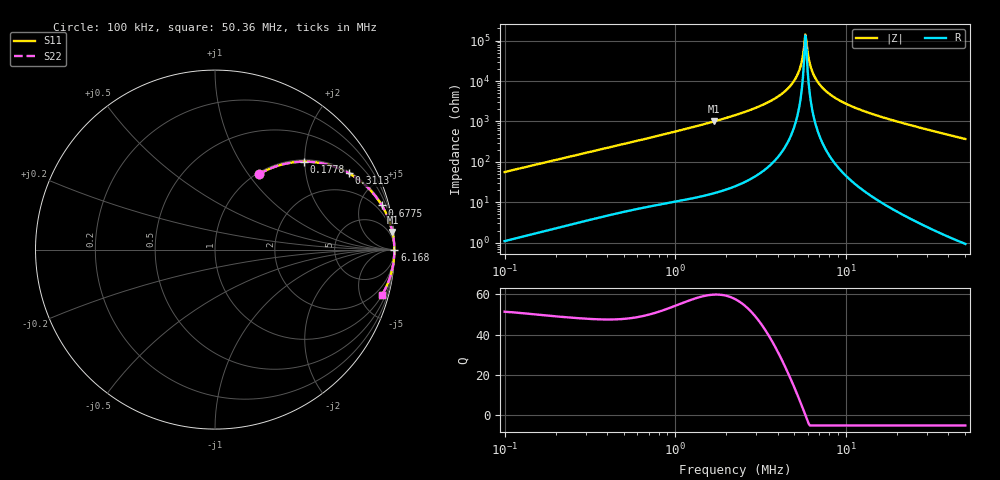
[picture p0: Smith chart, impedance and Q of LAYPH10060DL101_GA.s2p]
! LAYPH10060DL101_GA  S-PARAMETER MODEL  ( General Type )
! Model Generated by TAIYO YUDEN Corporation (http://www.ty-top.com)
! Version 3.0
! TAIYO YUDEN Control No. 180828NI43SB-FBB
! Copyright(c) 2017 TAIYO YUDEN CO.,LTD. All Rights Reserved.
! Product Description (link to TY-COMPAS)
! https://ds.yuden.co.jp/TYCOMPAS/or/detail?pn=LAYPH10060DL101MGA&u=M
! Products Name : Inductors
! Characteristics :
!  Inductance : 100 uH , SRF(min) : -Hz , DC Resistance(max) : 0.203 Ohm
!  Rated Current : Saturation :1.4 A , Temp Rise : 0.93 A (25 degC)
!  Case Size : 10.1 x 10.0 / 0.398 x 0.394 [mm/inch] , Thickness : 6 / 0.236 [mm/inch]
!  (Conditions: Temperature = 25 degC , DC Bias Current/Voltage = 0A / 0V)
! External Node Assignments :
!  1  o---GGG---o  2
! GND o---------o GND
! Frequency Range : 0.1MHz  -  50.361429MHz  [ 402 STEP ]
# MHz S RI R 50
! Freq[MHz].  S11 Real  S11 Imag  S21 Real  S21 Imag  S12 Real  S12 Imag  S22 Real  S22 Imag
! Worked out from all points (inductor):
!   401 points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, 100 kHz to 50.36 MHz, reference 50 ohm
!   read as one part in series: L = 89.2 uH near 103.2 kHz
!   highest Q = 59.7 at 1.696 MHz (marker M1), where L = 94.4 uH
!   self-resonance near 5.796 MHz
!   S11 on the Smith chart (normalised r, x): 100 kHz: 1.02, +1.12; 177.8 kHz: 1.04, +1.99; 311.3 kHz: 1.07, +3.46; 677.5 kHz: 1.15, +7.52; 6.168 MHz: open; 50.36 MHz: 1.02, -7.37
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0.1  0.2445 0.4202  0.7555 -0.4202  0.7555 -0.4202  0.2445 0.4202
0.177805  0.497 0.49  0.503 -0.49  0.503 -0.49  0.497 0.49
0.283532  0.7094 0.4437  0.2906 -0.4437  0.2906 -0.4437  0.7094 0.4437
0.311267  0.7452 0.4254  0.2548 -0.4254  0.2548 -0.4254  0.7452 0.4254
0.677478  0.9297 0.2457  0.0703 -0.2457  0.0703 -0.2457  0.9297 0.2457
0.803902  0.9488 0.2109  0.0512 -0.2109  0.0512 -0.2109  0.9488 0.2109
1.696112  0.9886 0.0981  0.0114 -0.0981  0.0114 -0.0981  0.9886 0.0981
2.279315  0.9942 0.068  0.00585 -0.068  0.00585 -0.068  0.9942 0.068
3.523312  0.9981 0.0331  0.00193 -0.0331  0.00193 -0.0331  0.9981 0.0331
4.589763  0.999 0.0152  0.000953 -0.0152  0.000953 -0.0152  0.999 0.0152
5.279436  0.9993 0.00616  0.000722 -0.00616  0.000722 -0.00616  0.9993 0.00616
5.446255  0.9993 0.00418  0.000694 -0.00418  0.000694 -0.00418  0.9993 0.00418
5.70642  0.9993 0.00122  0.000668 -0.00122  0.000668 -0.00122  0.9993 0.00122
5.795875  0.9993 0.000234  0.000664 -0.000234  0.000664 -0.000234  0.9993 0.000234
5.979013  0.9993 -0.00174  0.00066 0.00174  0.00066 0.00174  0.9993 -0.00174
6.167937  0.9993 -0.00371  0.000666 0.00371  0.000666 0.00371  0.9993 -0.00371
6.362832  0.9993 -0.00569  0.000679 0.00569  0.000679 0.00569  0.9993 -0.00569
7.094751  0.9992 -0.0127  0.000791 0.0127  0.000791 0.0127  0.9992 -0.0127
8.684711  0.9987 -0.0261  0.00129 0.0261  0.00129 0.0261  0.9987 -0.0261
11.67092  0.9971 -0.0477  0.00287 0.0477  0.00287 0.0477  0.9971 -0.0477
18.04064  0.9917 -0.0875  0.0083 0.0875  0.0083 0.0875  0.9917 -0.0875
50.36143  0.9309 -0.2524  0.0691 0.2524  0.0691 0.2524  0.9309 -0.2524
